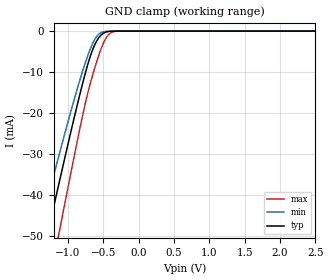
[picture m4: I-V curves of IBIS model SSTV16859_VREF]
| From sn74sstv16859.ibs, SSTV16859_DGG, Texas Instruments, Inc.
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[Model]   SSTV16859_VREF
Model_type  Input
Vinl = 1.15
Vinh = 1.35
| variable   typ   min   max
C_comp   4.38pF   2.08pF   5.75pF
[Temperature Range]   40   85   0
| Ambient temperature   25   70   0
[Voltage range]   2.5   2.3   2.7
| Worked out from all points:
|   GND clamp passes 1 mA (typ) near -0.53 V on its own axis
[GND Clamp]
| SSTV16859_VREF
|   Voltage   I(typ)   I(min)   I(max)
-2.5V     -144.6mA   -125.3mA   -170.2mA
-1.415V   -59.27mA   -49.43mA   -74.73mA
-1.295V   -49.98mA   -41.36mA   -64.12mA
-1.255V   -46.9mA    -38.69mA   -60.59mA
-1.115V   -36.21mA   -29.49mA   -48.24mA
-885mV    -19.17mA   -15.06mA   -28.22mA
-730mV    -8.736mA   -6.467mA   -15.8mA
-635mV    -3.871mA   -2.47mA    -9.784mA
-535mV    -1.041mA   -423.2uA   -4.484mA
-435mV    -130.8uA   -40.84uA   -1.067mA
-310mV    -3.568uA   -1.316uA   -43.83uA
2.5V      594.9pA    425.2pA    6.012nA
